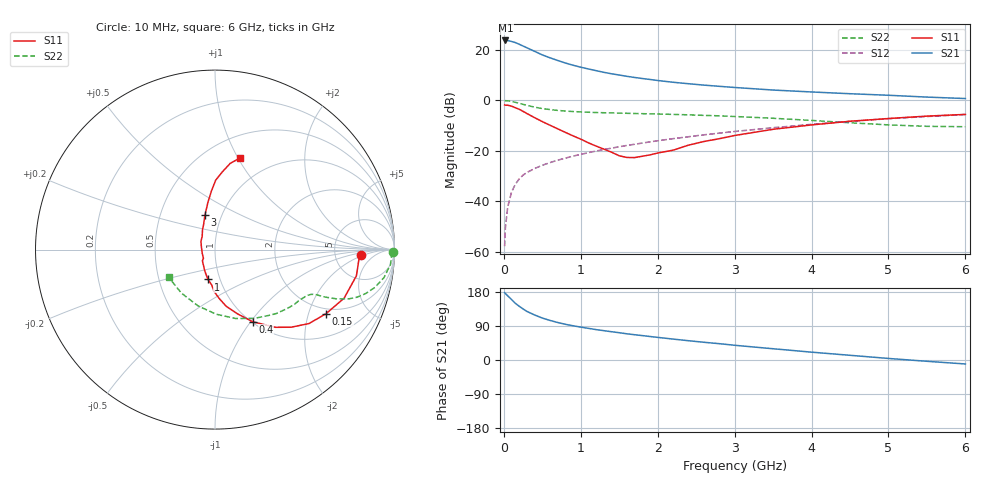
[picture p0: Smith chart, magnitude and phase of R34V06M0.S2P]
! SIEMENS Small Signal Semiconductors
! BFR181
! Si NPN RF Bipolar Junction Transistor in SOT23
! VCE = 4 V  IC = 6 mA
! Common Emitter S-Parameters:  May  1996
# GHz  S  MA  R  50
!  f  S11  S21  S12  S22
! GHz  MAG  ANG  MAG  ANG  MAG  ANG  MAG  ANG
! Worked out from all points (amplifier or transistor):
!   36 points, 10 MHz to 6 GHz, reference 50 ohm
!   highest |S21| = 23.7 dB at 20 MHz (marker M1)
!   |S21| within 3 dB of that: start of sweep to 307.4 MHz
!   unconditionally stable (mu >= 1): 1.046 GHz to 2.885 GHz
!   at 250 MHz: K = 0.46, MSG = 25.5 dB, |S12| = -29.6 dB
!   at 1.4 GHz: K = 1.05, MAG = 13.4 dB, |S12| = -18.9 dB
!   at 6 GHz: K = 0.86, MSG = 3.2 dB, |S12| = -5.6 dB
!   S11 on the Smith chart (normalised r, x): 10 MHz: 9.41, -1.66; 150 MHz: 1.79, -2.62; 400 MHz: 1.01, -1.03; 1 GHz: 0.88, -0.30; 3 GHz: 0.83, +0.34; 6 GHz: 0.72, +1.02
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0.01  0.8132 -2.1  15.33 177.6  0.0013 96.2  0.9906 -0.9
0.02  0.8033 -4.2  15.34 175.4  0.003 87.8  0.9847 -2.0
0.05  0.8013 -10.5  15.32 169.4  0.0077 86.6  0.9809 -4.9
0.1  0.7686 -20.6  14.66 159.6  0.0153 80.4  0.9544 -9.4
0.15  0.7143 -30.0  13.92 149.5  0.0219 75.0  0.9155 -13.3
0.2  0.6663 -38.2  12.91 141.8  0.0279 71.5  0.8738 -16.3
0.25  0.6061 -45.5  11.9 134.7  0.0332 68.9  0.8354 -18.5
0.3  0.5487 -52.1  10.99 128.2  0.0373 68.0  0.797 -20.1
0.4  0.4545 -62.3  9.347 118.8  0.0448 65.6  0.734 -22.0
0.5  0.38 -70.6  7.941 110.7  0.0519 64.9  0.6884 -22.9
0.6  0.322 -78.8  6.957 104.4  0.0587 65.0  0.6573 -23.5
0.8  0.2323 -91.4  5.488 94.2  0.0719 65.0  0.6146 -24.1
1  0.1708 -103.2  4.532 86.8  0.0853 65.6  0.5902 -25.0
1.1  0.1442 -110.9  4.184 83.5  0.0923 65.8  0.5822 -25.7
1.3  0.1085 -126.2  3.59 77.4  0.1066 65.9  0.5689 -27.1
1.6  0.0741 -163.7  2.99 69.1  0.1282 65.7  0.5548 -29.7
2.2  0.1033 133.6  2.283 55.2  0.1746 63.5  0.5275 -37.0
3  0.2017 106.0  1.8 38.9  0.2422 58.4  0.4795 -49.4
3.5  0.2675 98.4  1.601 29.7  0.2875 54.2  0.4422 -60.0
4.5  0.386 89.5  1.354 12.4  0.3844 43.9  0.36 -89.0
5.5  0.4879 80.0  1.161 -3.4  0.4795 31.3  0.3063 -127.7
6  0.5276 74.9  1.087 -10.5  0.5233 24.3  0.3007 -149.3
